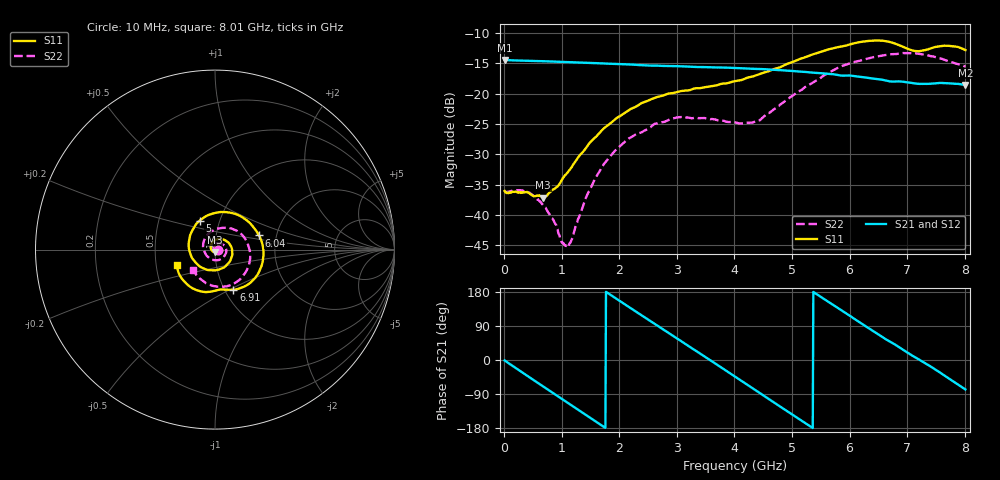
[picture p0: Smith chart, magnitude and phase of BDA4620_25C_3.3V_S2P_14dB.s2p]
!Agilent Technologies,E5071B,MY42404982,A.09.10
!Date: Wed May 06 08:51:32 2026
!Data & Calibration Information:
!Freq	S11:SOLT2(ON)	S21:SOLT2(ON)	S12:SOLT2(ON)	S22:SOLT2(ON)
# Hz S RI R 50
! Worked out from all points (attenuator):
!   801 points, 10 MHz to 8.01 GHz, reference 50 ohm
!   highest |S21| = -14.42 dB at 10 MHz (marker M1); lowest = -18.5 dB at 8.01 GHz (marker M2)
!   lowest |S11| = -37.1 dB at 680 MHz (marker M3), VSWR 1.03, Z = 49.7 - j1.36 ohm
!   |S11| at or under -10 dB: start of sweep to end of sweep
!   |S22| runs from -45.1 to -13.3 dB; largest |S21 - S12| = 0.00077
!   S11 on the Smith chart (normalised r, x): 10 MHz: 1.03, -0.00; 5 GHz: 0.80, +0.27; 6.04 GHz: 1.62, +0.27; 6.91 GHz: 1.10, -0.52; 8.01 GHz: 0.64, -0.12
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1e7  0.0157 -0.00109  0.1901 -0.00406  0.1904 -0.00406  0.0156 -0.000634
4.2e8  0.00891 -0.0124  0.1359 -0.1286  0.1361 -0.1288  0.0137 -0.0069
6.8e8  -0.00257 -0.0137  0.0638 -0.1744  0.0637 -0.1746  0.00782 -0.0092
1.08e9  -0.0218 0.00124  -0.0642 -0.1712  -0.0645 -0.1714  -0.0044 -0.00341
1.16e9  -0.0232 0.00727  -0.0875 -0.1598  -0.0878 -0.16  -0.00604 -0.000517
1.35e9  -0.0236 0.0224  -0.1342 -0.1212  -0.1344 -0.1213  -0.00819 0.00745
1.59e9  -0.0134 0.0419  -0.1704 -0.0551  -0.1705 -0.0551  -0.00604 0.0193
1.9e9  0.0155 0.0581  -0.172 0.0405  -0.1722 0.0406  0.00636 0.0321
2.68e9  0.0948 0.00259  0.00284 0.1703  0.00304 0.1707  0.0543 0.018
3.4e9  0.0383 -0.1045  0.1587 0.0498  0.159 0.0497  0.0456 -0.0435
4.01e9  -0.0898 -0.0899  0.1179 -0.1131  0.118 -0.1134  -0.0227 -0.0535
4.42e9  -0.1446 0.00226  0.014 -0.1597  0.0139 -0.1598  -0.0594 -0.0097
5e9  -0.0858 0.1606  -0.124 -0.0917  -0.1243 -0.0918  -0.0359 0.0889
5.35e9  0.0262 0.209  -0.1496 -0.00385  -0.1497 -0.00384  0.0294 0.1191
5.66e9  0.1409 0.1869  -0.1268 0.0717  -0.127 0.0719  0.0986 0.1147
6.04e9  0.2456 0.0791  -0.0548 0.1298  -0.055 0.13  0.1729 0.0528
6.36e9  0.2666 -0.0616  0.021 0.1329  0.021 0.133  0.1961 -0.0264
6.68e9  0.1902 -0.19  0.0813 0.0975  0.0815 0.0977  0.1779 -0.1122
6.91e9  0.1023 -0.2238  0.1106 0.0605  0.1108 0.0607  0.1404 -0.1648
7.19e9  0.0281 -0.2225  0.1209 0.0052  0.1212 0.00529  0.0651 -0.2046
7.57e9  -0.0914 -0.229  0.1027 -0.0673  0.1029 -0.0673  -0.0396 -0.1915
8.01e9  -0.2118 -0.0878  0.0251 -0.1159  0.0253 -0.1161  -0.1224 -0.1143
